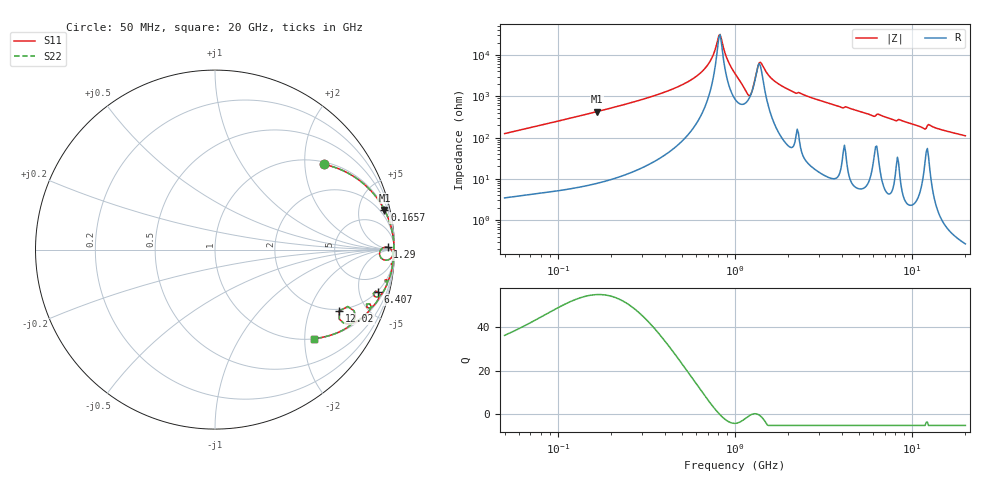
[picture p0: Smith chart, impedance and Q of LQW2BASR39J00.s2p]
!Murata Part Number: LQW2BASR39J00
!These Parameters are Measured in Series Mode Connection
!  o--[Z]--o
!Port1  Port2
!  o-------o
!Freq. Start=50[MHz] Stop=20[GHz], 401[Steps]
# Hz S RI R 50
!Freq.(Hz) S11(Real) S11(Imag) S21(Real) S21(Imag) S12(Real) S12(Imag) S22(Real) S22(Imag)
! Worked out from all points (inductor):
!   401 points, 50 MHz to 20 GHz, reference 50 ohm
!   read as one part in series: L = 395 nH near 51.52 MHz
!   highest Q = 54.7 at 165.7 MHz (marker M1), where L = 408 nH
!   self-resonance near 810.8 MHz
!   S11 on the Smith chart (normalised r, x): 50 MHz: 1.07, +2.50; 165.7 MHz: 1.16, +8.50; 1.29 GHz: 46, +16; 6.407 GHz: 1.82, -7.38; 12.02 GHz: 1.91, -3.23; 20 GHz: 1.01, -2.21
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5e7  0.6072 0.4747  0.3928 -0.4747  0.3928 -0.4747  0.6072 0.4747
1.364002e8  0.9186 0.2643  0.0814 -0.2643  0.0814 -0.2643  0.9186 0.2643
1.657227e8  0.9439 0.2212  0.0561 -0.2212  0.0561 -0.2212  0.9439 0.2212
3.721004e8  0.9899 0.0873  0.0101 -0.0873  0.0101 -0.0873  0.9899 0.0873
6.476653e8  0.9969 0.0254  0.00306 -0.0254  0.00306 -0.0254  0.9969 0.0254
7.30116e8  0.9972 0.0128  0.0028 -0.0128  0.0028 -0.0128  0.9972 0.0128
8.108264e8  0.9969 0.00138  0.00306 -0.00138  0.00306 -0.00138  0.9969 0.00138
8.354841e8  0.9967 -0.00206  0.00325 0.00206  0.00325 0.00206  0.9967 -0.00206
9.00459e8  0.9959 -0.0113  0.00412 0.0113  0.00412 0.0113  0.9959 -0.0113
1e9  0.9926 -0.0269  0.00744 0.0269  0.00744 0.0269  0.9926 -0.0269
1.196911e9  0.9244 -0.0459  0.0756 0.0459  0.0756 0.0459  0.9244 -0.0459
1.23331e9  0.9202 -0.00542  0.0798 0.00542  0.0798 0.00542  0.9202 -0.00542
1.289994e9  0.9616 0.0131  0.0384 -0.0131  0.0384 -0.0131  0.9616 0.0131
1.349283e9  0.982 0.000387  0.018 -0.000387  0.018 -0.000387  0.982 0.000387
1.390315e9  0.9877 -0.00805  0.0123 0.00805  0.0123 0.00805  0.9877 -0.00805
1.766834e9  0.9942 -0.05  0.00584 0.05  0.00584 0.05  0.9942 -0.05
2.728004e9  0.986 -0.1076  0.014 0.1076  0.014 0.1076  0.986 -0.1076
6.406762e9  0.9095 -0.2365  0.0905 0.2365  0.0905 0.2365  0.9095 -0.2365
7.442007e9  0.892 -0.3032  0.108 0.3032  0.108 0.3032  0.892 -0.3032
1.201863e10  0.6922 -0.3419  0.3078 0.3419  0.3078 0.3419  0.6922 -0.3419
1.295331e10  0.7694 -0.4038  0.2306 0.4038  0.2306 0.4038  0.7694 -0.4038
2e10  0.5502 -0.4963  0.4498 0.4963  0.4498 0.4963  0.5502 -0.4963
